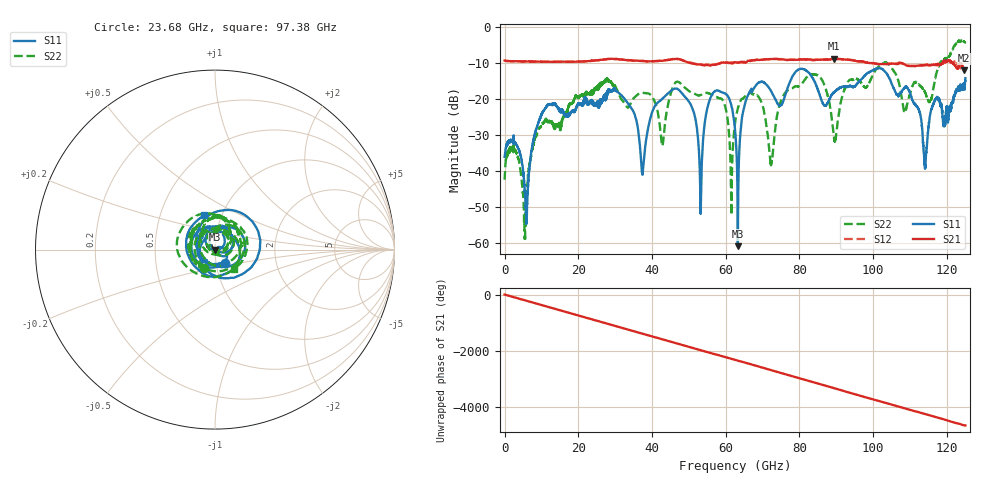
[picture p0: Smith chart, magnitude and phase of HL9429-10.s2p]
! 1/17/2024 3:29:39 PM
! H:\PROTOTYPE_DATA\110GHZ-ATTN\10DB\3091-2.S2P
! CHANNEL.1
! TR.MEASUREMENT
! CORRECTED.DATA
# GHZ S RI R 50.0
! FREQ.GHZ  S11RE  S11IM  S21RE  S21IM  S12RE  S12IM  S22RE  S22IM
!; PortSelection: Port_12
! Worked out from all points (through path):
!   5000 points, 25 MHz to 125 GHz, reference 50 ohm
!   highest |S21| = -8.89 dB at 89.45 GHz (marker M1); lowest = -12.1 dB at 124.6 GHz (marker M2)
!   group delay of S21, straight-line fit = 103 ps
!   lowest |S11| = -60.9 dB at 63.27 GHz (marker M3), VSWR 1.00, Z = 50 - j0.0903 ohm
!   |S11| at or under -10 dB: start of sweep to end of sweep
!   |S22| runs from -59.5 to -3.8 dB; largest |S21 - S12| = 0.14
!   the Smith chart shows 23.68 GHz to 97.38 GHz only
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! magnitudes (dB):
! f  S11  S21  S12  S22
! 25 MHz  -36.1  -9.4  -9.4  -42.5
! 2.975 GHz  -32.4  -9.6  -9.6  -34.6
! 5.575 GHz  -47.3  -9.6  -9.6  -59.5
! 10.7 GHz  -23.2  -9.7  -9.7  -26.5
! 20.88 GHz  -21.7  -9.6  -9.6  -18.9
! 31.5 GHz  -18.8  -9.1  -9.1  -19.8
! 37.45 GHz  -40.8  -9.5  -9.5  -18.3
! 41.7 GHz  -20.9  -9.5  -9.5  -24.4
! 50.02 GHz  -20.8  -10.0  -9.9  -17.8
! 53.17 GHz  -51.6  -10.5  -10.5  -19.0
! 56.83 GHz  -18.1  -10.6  -10.5  -19.1
! 61.48 GHz  -21.7  -10.1  -10.0  -47.4
! 62.52 GHz  -28.5  -9.8  -10.0  -26.8
! 63.27 GHz  -60.9  -10.0  -10.0  -22.6
! 66.15 GHz  -18.7  -9.4  -9.6  -18.6
! 72.35 GHz  -17.9  -8.9  -9.0  -37.7
! 83.35 GHz  -13.8  -9.1  -9.2  -13.2
! 89.45 GHz  -18.2  -8.9  -9.0  -31.6
! 104.2 GHz  -13.9  -10.3  -10.3  -10.3
! 114.1 GHz  -38.2  -10.6  -10.6  -18.3
! 124.6 GHz  -16.9  -12.1  -11.6  -4.1
! 125 GHz  -14.2  -11.7  -12.1  -4.3
